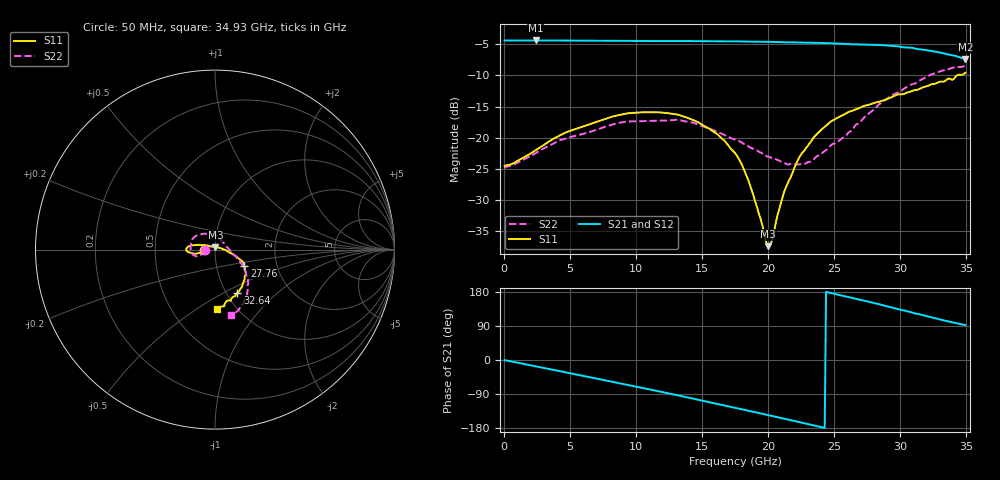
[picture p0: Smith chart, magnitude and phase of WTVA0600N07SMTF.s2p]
! 50 ohm 2-Port S-parameters measured by Modelithics Inc support@modelithics.com  Tampa, FL USA 813-866-6335 (February 2024)
! Smiths Interconnect,  6dB P/N: WTVA0600N07SMTF, Temperature: 75 C
! Board: 10 mil Rogers 4350B, Mounting Pad Dimensions: Length: 15 mils, Width: 25 mils, Gap: 40 mils.
# Hz S RI R 50
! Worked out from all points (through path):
!   352 points, 50 MHz to 34.93 GHz, reference 50 ohm
!   highest |S21| = -4.38 dB at 2.389 GHz (marker M1); lowest = -7.4 dB at 34.93 GHz (marker M2)
!   group delay of S21, straight-line fit = 21.3 ps
!   lowest |S11| = -37.4 dB at 20 GHz (marker M3), VSWR 1.03, Z = 50.2 + j1.33 ohm
!   |S11| at or under -10 dB: start of sweep to 34.29 GHz
!   |S22| runs from -24.9 to -8.5 dB; largest |S21 - S12| = 0.0071
!   S11 on the Smith chart (normalised r, x): 50 MHz: 0.89, -0.00; 27.76 GHz: 1.36, -0.25; 32.64 GHz: 1.12, -0.58; 34.93 GHz: 0.82, -0.61
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5e7  -0.0592 -8.73e-05  0.604 -0.00349  0.6035 -0.00337  -0.0567 -0.00188
2.389e9  -0.0778 -0.0153  0.579 -0.1722  0.5785 -0.172  -0.0714 -0.0227
5.8715e9  -0.1196 -0.0222  0.4543 -0.3957  0.4537 -0.3954  -0.0994 -0.0377
9.354e9  -0.1566 -0.00903  0.2461 -0.5463  0.2454 -0.5456  -0.134 -0.0136
1.1742e10  -0.1596 0.00461  0.0744 -0.5928  0.073 -0.5923  -0.1344 0.0259
1.4727e10  -0.1308 0.0227  -0.1549 -0.5762  -0.1554 -0.5754  -0.0992 0.0795
1.612e10  -0.1043 0.026  -0.2563 -0.5371  -0.257 -0.5361  -0.0699 0.0871
1.7513e10  -0.0706 0.0244  -0.3503 -0.4801  -0.3504 -0.4791  -0.0379 0.0886
1.8508e10  -0.0392 0.0223  -0.4095 -0.4265  -0.4097 -0.4255  -0.0119 0.084
2.00005e10  0.00209 0.0133  -0.485 -0.3337  -0.4844 -0.3332  0.017 0.0681
2.0299e10  0.0094 0.0119  -0.498 -0.3127  -0.4975 -0.3122  0.0209 0.0653
2.0697e10  0.0207 0.0114  -0.5129 -0.2843  -0.5125 -0.2834  0.0273 0.0604
2.1294e10  0.0385 0.0047  -0.5316 -0.2409  -0.531 -0.2403  0.0347 0.0516
2.23885e10  0.0699 -0.00864  -0.5591 -0.1596  -0.559 -0.1577  0.0508 0.034
2.33835e10  0.0956 -0.0234  -0.5729 -0.0802  -0.5723 -0.0801  0.0637 0.0167
2.47765e10  0.1278 -0.0452  -0.5729 0.0337  -0.5722 0.0348  0.0871 -0.00809
2.5871e10  0.1448 -0.0586  -0.5526 0.1215  -0.5521 0.1208  0.1 -0.0249
2.77615e10  0.1628 -0.089  -0.4948 0.2572  -0.4925 0.26  0.1431 -0.0731
2.91545e10  0.1688 -0.1199  -0.423 0.3498  -0.4189 0.3534  0.1716 -0.1237
3.1045e10  0.1596 -0.1797  -0.2882 0.4367  -0.2875 0.4362  0.1802 -0.2021
3.2637e10  0.1244 -0.2411  -0.1693 0.4612  -0.1663 0.4616  0.1641 -0.2848
3.49255e10  0.0113 -0.3318  -0.0159 0.4273  -0.0154 0.4265  0.0868 -0.3669
